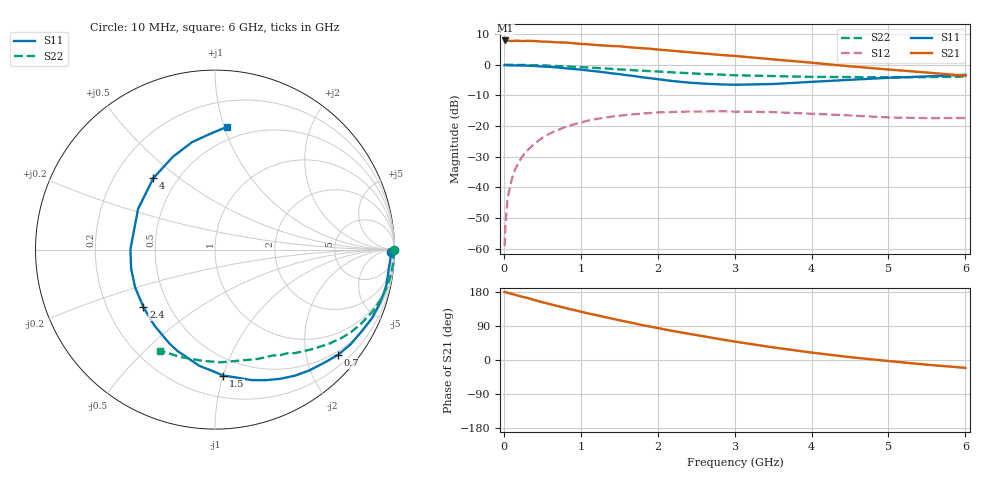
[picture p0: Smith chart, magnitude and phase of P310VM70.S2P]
! SIEMENS Small Signal Semiconductors
! BFP181
! Si NPN RF Bipolar Junction Transistor in SOT143
! VCE = 10 V  IC = 0.7 mA
! Common Emitter S-Parameters:  March  1996
# GHz  S  MA  R  50
!  f  S11  S21  S12  S22
! GHz  MAG  ANG  MAG  ANG  MAG  ANG  MAG  ANG
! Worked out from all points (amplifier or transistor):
!   36 points, 10 MHz to 6 GHz, reference 50 ohm
!   highest |S21| = 7.9 dB at 20 MHz (marker M1)
!   |S21| within 3 dB of that: start of sweep to 2.018 GHz
!   unconditionally stable (mu >= 1): 3.622 GHz to end of sweep
!   at 250 MHz: K = 0.07, MSG = 18.6 dB, |S12| = -29.6 dB
!   at 1.4 GHz: K = 0.44, MSG = 11.5 dB, |S12| = -16.9 dB
!   at 6 GHz: K = 1.35, MAG = 3.4 dB, |S12| = -17.4 dB
!   S11 on the Smith chart (normalised r, x): 10 MHz: 67, -47; 700 MHz: 0.42, -2.65; 1.5 GHz: 0.36, -1.00; 2.4 GHz: 0.36, -0.31; 4 GHz: 0.37, +0.41; 6 GHz: 0.39, +1.02
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0.01  0.9803 -0.8  2.454 179.4  0.0011 71.2  0.9983 -0.2
0.02  0.9863 -1.2  2.488 179.5  0.0023 77.6  0.9978 -0.6
0.05  0.9794 -2.6  2.481 177.3  0.0068 90.8  0.996 -1.5
0.1  0.9747 -6.0  2.428 174.6  0.0131 85.2  0.9959 -2.8
0.15  0.9739 -9.0  2.465 171.8  0.0201 83.6  0.9953 -4.3
0.2  0.9749 -11.8  2.453 169.0  0.0264 81.9  0.9928 -5.7
0.3  0.9666 -17.6  2.453 164.2  0.0394 77.7  0.9884 -8.6
0.4  0.9546 -23.5  2.437 157.9  0.0521 73.6  0.9827 -11.4
0.6  0.9215 -34.9  2.364 147.4  0.0758 65.7  0.9647 -16.7
0.7  0.9027 -40.5  2.311 142.3  0.0862 62.0  0.9519 -19.4
0.8  0.875 -46.3  2.302 137.3  0.0966 58.2  0.9407 -21.9
1.1  0.8058 -63.3  2.157 122.6  0.123 47.7  0.9 -28.9
1.5  0.703 -86.3  2.004 105.0  0.1474 35.6  0.8403 -37.2
1.8  0.6231 -103.9  1.859 92.0  0.1598 28.1  0.7991 -42.4
2.2  0.5412 -128.7  1.687 76.4  0.1695 18.6  0.7489 -49.2
2.4  0.5117 -141.2  1.602 69.3  0.1727 14.3  0.7288 -52.3
3  0.4714 179.8  1.392 48.6  0.1721 3.9  0.6728 -61.2
3.5  0.4848 152.1  1.224 33.3  0.1688 -2.7  0.6538 -68.7
4  0.5259 130.8  1.079 19.6  0.159 -7.6  0.6334 -77.6
4.5  0.568 114.4  0.943 7.5  0.1488 -11.1  0.629 -87.4
5.5  0.6455 92.4  0.746 -12.4  0.1346 -8.6  0.6287 -108.0
6  0.686 84.6  0.662 -20.7  0.1355 -6.5  0.6409 -118.7
